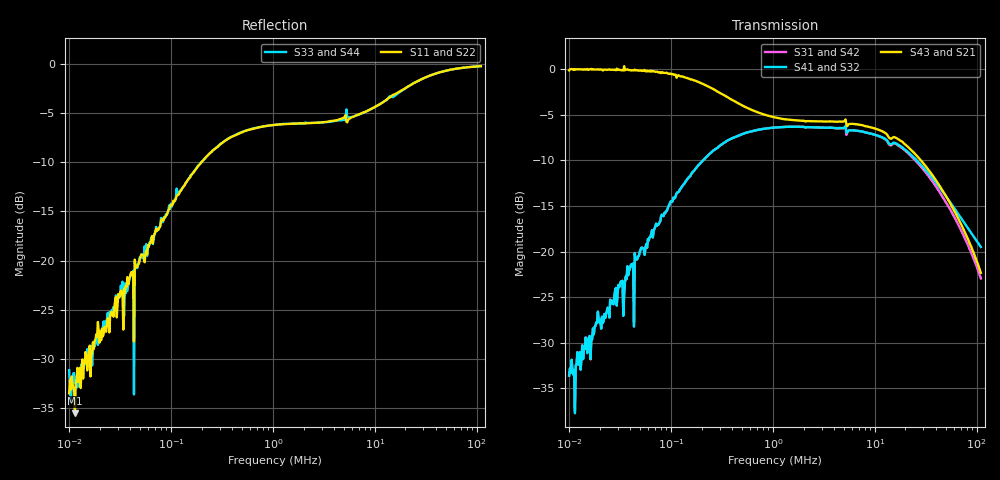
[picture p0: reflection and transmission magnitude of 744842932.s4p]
! Touchstone file was created by TriD Version 2018.1.1 (64-bit) (04.05.2018)
! (C) EMCoS 1999-2018
! Project : TRID_WE_CMB_NiZn_S_744_842_932_Task 1\Task 1.in
! Date  : 2018-06-26  02:18:53
# HZ S RI R  50.00
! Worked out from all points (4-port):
!   503 points, 10 kHz to 110 MHz, reference 50 ohm
!   strongest paths, dB at 10 kHz, 101.6 kHz, 1.05 MHz, 10.85 MHz, 110 MHz:
!     S43: -0.2, -0.5, -5.3, -6.7, -22.3
!     S21: 0.0, -0.5, -5.3, -6.6, -22.4
!     S41: -33.6, -14.6, -6.4, -7.3, -19.5
!     S32: -33.6, -14.6, -6.4, -7.3, -19.5
!     S31: -33.6, -14.6, -6.4, -7.3, -22.9
!     S42: -33.6, -14.6, -6.4, -7.4, -24.0
!   lowest |S11| = -35.5 dB at 11.4 kHz (marker M1), VSWR 1.03, Z = 48.8 - j1.17 ohm
!   |S11| at or under -10 dB: start of sweep to 199.1 kHz
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10000  0.00405 0.0208  0.996 -0.0208  0.0209 0.0189  -0.0209 -0.0188
       0.996 -0.0208  0.00403 0.0208  -0.0209 -0.0188  0.0209 0.0188
       0.00417 0.0205  -0.00415 -0.0205  0.0194 0.0199  0.9806 -0.0198
       -0.00417 -0.0205  0.00416 0.0206  0.9806 -0.0199  0.0194 0.0198
11404  -0.0117 -0.012  1.012 0.012  0.0126 0.0206  -0.0127 -0.0206
       1.012 0.0124  -0.0121 -0.0124  -0.0127 -0.0206  0.0128 0.0206
       -0.0104 -0.00851  0.0106 0.00851  0.0117 0.0209  0.9882 -0.0209
       0.0102 0.00806  -0.0103 -0.00805  0.9884 -0.0209  0.0118 0.0209
144470  0.1352 0.216  0.8648 -0.2162  0.135 0.2091  -0.135 -0.2089
        0.8649 -0.2166  0.1351 0.2166  -0.1351 -0.2094  0.1351 0.2094
        0.135 0.21  -0.135 -0.2101  0.1351 0.2159  0.8649 -0.2159
        -0.135 -0.2095  0.135 0.2097  0.8651 -0.2156  0.135 0.2153
685360  0.4414 0.1681  0.5585 -0.1686  0.4414 0.1376  -0.4413 -0.1372
        0.5583 -0.1687  0.4416 0.1683  -0.4413 -0.1371  0.4414 0.1373
        0.4407 0.138  -0.4406 -0.1377  0.4423 0.1677  0.5576 -0.1681
        -0.4405 -0.1375  0.4405 0.1378  0.5576 -0.1683  0.4424 0.1679
1.4058e7  0.6307 0.2388  0.3676 -0.248  0.3434 -0.2272  -0.3416 0.2328
          0.3703 -0.2503  0.6298 0.2412  -0.3444 0.2352  0.3442 -0.2301
          0.3256 -0.2008  -0.3248 0.2052  0.6501 0.2124  0.349 -0.2203
          -0.3269 0.209  0.3277 -0.2026  0.3512 -0.2246  0.6481 0.2142
4.119e7  0.8792 0.1827  0.1184 -0.2073  0.1013 -0.1965  -0.099 0.2103
         0.1185 -0.2076  0.8804 0.1803  -0.0991 0.2107  0.1001 -0.1945
         0.1011 -0.1963  -0.0988 0.21  0.8794 0.1825  0.1182 -0.207
         -0.0989 0.2104  0.0999 -0.1942  0.1184 -0.2074  0.8806 0.18
1.1e8  0.9727 0.00873  0.022 -0.0729  0.0087 -0.0706  -0.00379 0.1057
       0.022 -0.0728  0.9733 -0.000373  -0.00379 0.1057  0.00802 -0.0623
       0.00864 -0.0707  -0.00374 0.1058  0.9728 0.00901  0.0219 -0.0731
       -0.00375 0.1058  0.00799 -0.0624  0.0219 -0.0731  0.9734 -0.000113
